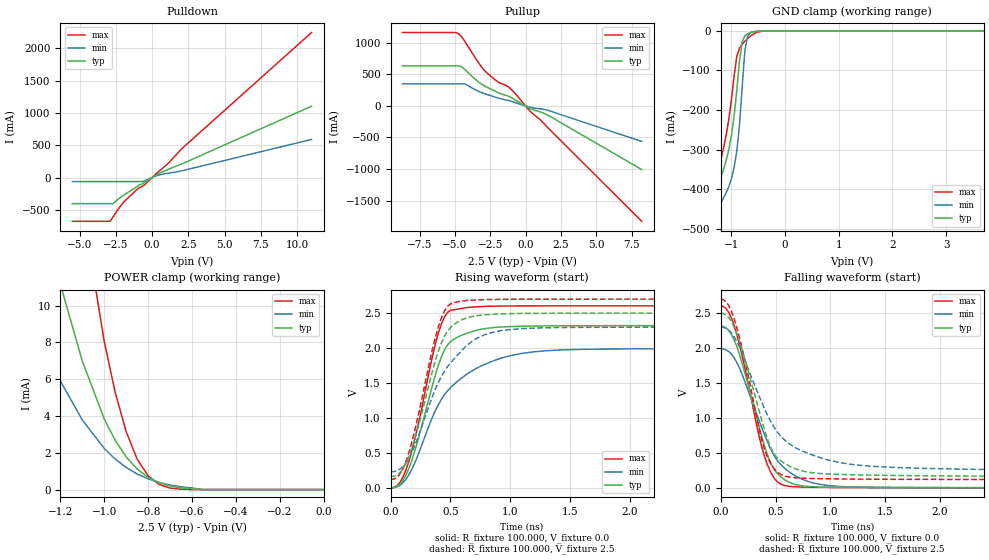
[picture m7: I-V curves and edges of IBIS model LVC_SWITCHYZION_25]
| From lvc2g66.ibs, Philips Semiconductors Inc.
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|   Model LVC_SWITCHYZION_25
[Model]   LVC_SWITCHYZION_25
Model_type   I/O
Polarity   Non-Inverting
Enable   Active-High
Vinl  =  0.7V
Vinh  =  1.7V
Vmeas =  1.25V
Cref  =  30.0pF
Rref  =  0.5k
Vref  =  0.0V
C_comp   7.87pF   4.15pF   10.52pF
[Model Spec]
| Note: The input and output voltage ratings may be exceeded if the input and
|   output current ratings are observed (please refer to the data sheet)
|   Subparameter   typ   min   max
| Thresholds
Vinh   1.7   1.7   1.7
Vinl   0.7   0.7   0.7
| Overshoot
S_overshoot_high   6.5   6.5   6.5   | Static overshoot
S_overshoot_low   -0.5   -0.5   -0.5
D_overshoot_high   7.2   7.2   7.2   | Dynamic overshoot
D_overshoot_low   -0.95   -0.9   -1.0
D_overshoot_time   3n   3n   3n
| Timing Thresholds
Vmeas   1.25   1.15   1.35
|Ambient temperature:   25   85   -40
[Temperature Range]   30   90   -35
[Voltage Range]   2.5V   2.3V   2.7V
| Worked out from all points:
|   slope of the pulldown table from 0 to 0.375 V, typ, clamps not added: 7.27 ohm
|   slope of the pullup table from 0 to 0.375 V, typ, clamps not added: 8.36 ohm
|   GND clamp passes 1 mA (typ) near -0.48 V on its own axis
|   POWER clamp passes 1 mA (typ) near -0.84 V on its own axis
|   rising waveform, R_fixture 100.000, V_fixture 0.0: 20-80 % time 230ps typ, 398ps min, 202ps max; typ from 0 V to 2.32 V
|   rising waveform, R_fixture 100.000, V_fixture 2.5: 20-80 % time 226ps typ, 342ps min, 205ps max; typ from 0.162 V to 2.5 V
|   falling waveform, R_fixture 100.000, V_fixture 0.0: 20-80 % time 246ps typ, 311ps min, 221ps max; typ from 2.31 V to 0 V
|   falling waveform, R_fixture 100.000, V_fixture 2.5: 20-80 % time 259ps typ, 408ps min, 219ps max; typ from 2.5 V to 0.162 V
|Process Range   nominal   slow   fast
[Pulldown]
| voltage   I(typ)   I(min)   I(max)
-5.5V     -403.3mA   -62.78mA   -677.3mA
-2.9V     -403.3mA   -62.78mA   -677.3mA
-2.7V     -403.3mA   -62.78mA   -608.7mA
-2.3V     -329.1mA   -62.78mA   -477.5mA
-1.9V     -262.6mA   -62.78mA   -366.6mA
-950mV    -124.6mA   -62.78mA   -167.2mA
-650mV    -93.52mA   -60.62mA   -132mA
700mV     88.44mA    51.42mA    140.9mA
1V        116.3mA    63.37mA    196.4mA
2.2V      226.2mA    112.4mA    477mA
11V       1.104A     589.6mA    2.245A
[Pullup]
| voltage   I(typ)   I(min)   I(max)
-8.7V     636mA      351.5mA    1.164A
-4.9V     636mA      351.5mA    1.164A
-4.7V     636mA      351.5mA    1.139A
-4.3V     578.7mA    351.5mA    1.024A
-3.5V     412.6mA    250.6mA    743.5mA
-2.9V     316.8mA    194.4mA    559.6mA
-1.9V     206.5mA    123.6mA    373.5mA
-1.1V     144.3mA    80.5mA     281.4mA
400mV     -47.73mA   -24.77mA   -101.3mA
1V        -92.13mA   -44.66mA   -212.8mA
1.8V      -174.2mA   -84.37mA   -395.9mA
8.2V      -1.008A    -562mA     -1.829A
[GND_clamp]
| voltage   I(typ)   I(min)   I(max)
-5.5V     -5.602A    -5.222A    -6.266A
-1.4V     -522.8mA   -578.4mA   -487.1mA
-1.35V    -476.5mA   -532.5mA   -440.1mA
-1.3V     -432.2mA   -488.9mA   -394.8mA
-1.05V    -299.9mA   -393.2mA   -224mA
-900mV    -150mA     -302.9mA   -64.41mA
-850mV    -76.11mA   -238.1mA   -43.53mA
-800mV    -27.59mA   -141.5mA   -33.92mA
-750mV    -12.16mA   -50.28mA   -26.3mA
-700mV    -7.405mA   -14.01mA   -19.54mA
-600mV    -3.216mA   -2.246mA   -8.918mA
5.5V      766pA      6.791nA    76.23pA
[POWER_clamp]
| voltage   I(typ)   I(min)   I(max)
-8.7V     6.914A     6.943A     6.957A
-1.4V     22.15mA    14.06mA    48.9mA
-1.3V     16.24mA    8.888mA    36.12mA
-1.2V     11.15mA    5.9mA      24.84mA
-1.1V     6.976mA    3.781mA    15.37mA
-1V       3.837mA    2.237mA    8.041mA
-950mV    2.675mA    1.66mA     5.274mA
-900mV    1.776mA    1.202mA    3.147mA
-850mV    1.119mA    848.3uA    1.659mA
-800mV    668.7uA    584.2uA    749.2uA
-650mV    92.42uA    154.2uA    20.53uA
0V        0A         0A         0A
[Ramp]
| variable   typ   min   max
dV/dt_r   1.390V/229.857ps   1.195V/398.533ps   1.562V/201.993ps
dV/dt_f   1.403V/259.490ps   1.241V/407.920ps   1.548V/218.870ps
R_load = 100.000
[Rising Waveform]
R_fixture   = 100.000
V_fixture   = 0.0
V_fixture_min = 0.0
V_fixture_max = 0.0
| time   V(typ)   V(min)   V(max)
0s        142.7fV    6.687pV    21.09fV
75ps      48.44mV    32.29mV    70.02mV
125ps     171.9mV    114mV      239.6mV
200ps     513.1mV    348.2mV    677.6mV
400ps     1.756V     1.191V     2.217V
450ps     1.97V      1.329V     2.441V
525ps     2.122V     1.473V     2.548V
900ps     2.298V     1.842V     2.6V
1.4ns     2.318V     1.971V     2.604V
8.8ns     2.316V     1.991V     2.603V
[Rising Waveform]
R_fixture   = 100.000
V_fixture   = 2.5
V_fixture_min = 2.3
V_fixture_max = 2.7
| time   V(typ)   V(min)   V(max)
0s        161.6mV    230.5mV    119.7mV
75ps      210.8mV    263.6mV    190.5mV
150ps     434.1mV    414.9mV    487.6mV
350ps     1.668V     1.306V     1.982V
425ps     2.076V     1.593V     2.432V
475ps     2.24V      1.731V     2.594V
575ps     2.387V     1.927V     2.666V
825ps     2.48V      2.212V     2.694V
1.3ns     2.497V     2.29V      2.699V
8.8ns     2.5V       2.3V       2.7V
[Falling Waveform]
R_fixture   = 100.000
V_fixture   = 0.0
V_fixture_min = 0.0
V_fixture_max = 0.0
| time   V(typ)   V(min)   V(max)
0s        2.315V     1.992V     2.602V
75ps      2.248V     1.948V     2.506V
150ps     2.008V     1.784V     2.177V
350ps     879.4mV    965mV      741.5mV
425ps     477.8mV    664.2mV    335.4mV
500ps     238.6mV    428.8mV    113.3mV
600ps     100.1mV    257.7mV    28.47mV
850ps     14.75mV    68.84mV    8.135mV
1.3ns     5.751mV    9.447mV    3.374mV
8.8ns     9.626uV    162.2uV    64.79nV
[Falling Waveform]
R_fixture   = 100.000
V_fixture   = 2.5
V_fixture_min = 2.3
V_fixture_max = 2.7
| time   V(typ)   V(min)   V(max)
0s        2.5V       2.3V       2.7V
75ps      2.433V     2.253V     2.603V
150ps     2.193V     2.085V     2.276V
350ps     1.105V     1.316V     844.4mV
425ps     705.6mV    1.048V     445.9mV
500ps     458.4mV    834.4mV    250.5mV
625ps     313.5mV    631.2mV    154.8mV
1.1ns     191.5mV    357.9mV    127.2mV
1.7ns     175.4mV    285.8mV    121.9mV
8.8ns     161.6mV    231.3mV    119.7mV
